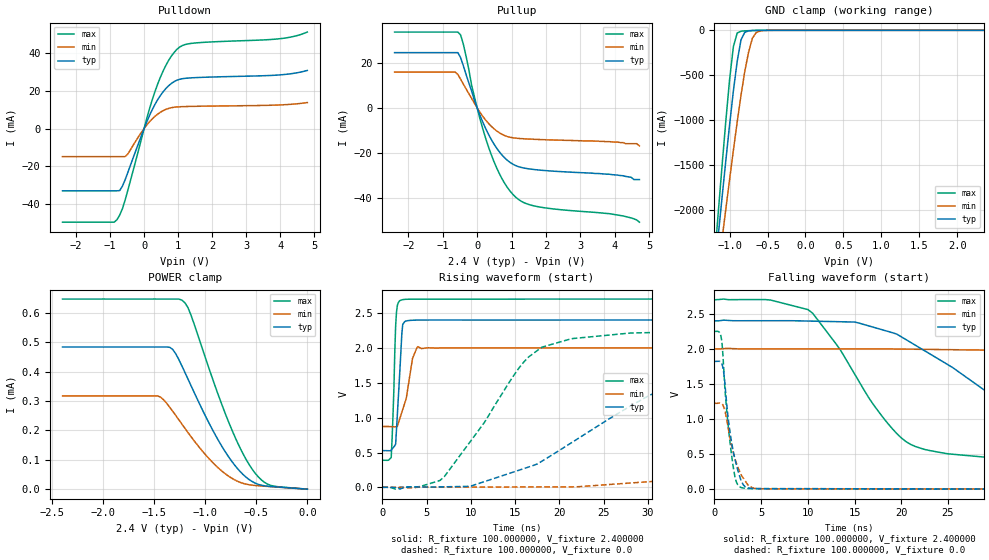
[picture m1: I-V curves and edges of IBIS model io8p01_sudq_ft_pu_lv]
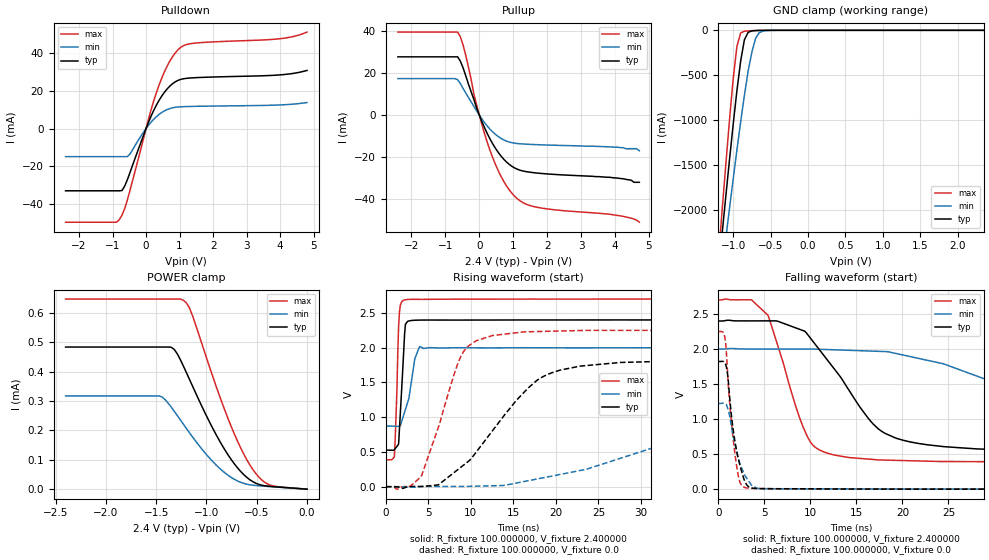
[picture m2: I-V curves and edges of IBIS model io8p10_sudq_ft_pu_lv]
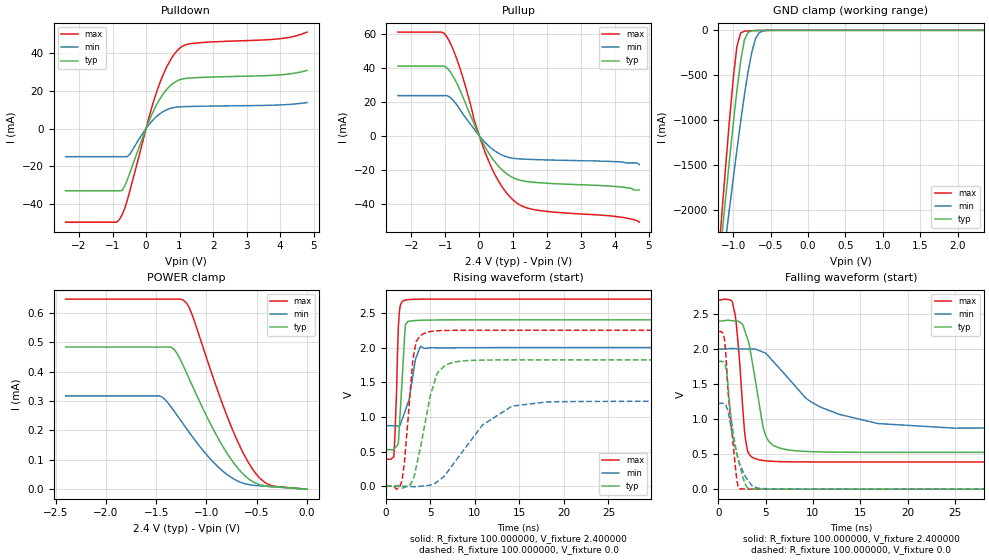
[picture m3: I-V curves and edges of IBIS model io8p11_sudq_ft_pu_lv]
|   stm32f0_444_ufqfpn32 IBIS Model
[IBIS ver]   4.2
[File name]  stm32f0_444_ufqfpn32.ibs
[File Rev]   1.0
[Date]   15-5-2013
[Source] Data Created at STMicroelectronics
[Notes]   File originated from ELDO simulations.
[Disclaimer]  This information is for modeling purpose only and is
   not guaranted. The information is subject to change without
   notice.
[Copyright] Copyright 2015 STMicroelectronics Inc.
[Component] stm32f0_444_ufqfpn32
[Manufacturer] STMicroelectronics
[Package]
| variable   typ   min   max
R_pkg   0.0   NA   NA
L_pkg   0.0H   NA   NA
C_pkg   0.0F   NA   NA
[Pin] signal_name  model_name   R_pin   L_pin   C_pin
0   VSS_VSSA   GND   NA   NA   NA
1   VDD   POWER   0.03449   2.11E-09   6E-14
2   PF0   io8p_sudq_ft   0.029020556   1.54333E-09   3.22222E-14
3   PF1   io8p_sudq_ft   0.025738889   1.20333E-09   1.55556E-14
4   NRST  ioreset_tc_v33   0.024645   1.09E-09   1E-14
5   VDDA  POWER   0.024645   1.09E-09   1E-14
6   PA0   io8p_sudq_ft   0.025738889   1.20333E-09   1.55556E-14
7   PA1   io8p_sudq_ft   0.029020556   1.54333E-09   3.22222E-14
8   PA2   io8p_sudq_ft   0.03449   2.11E-09   6E-14
9   PA3   io8p_sudq_ft   0.03449   2.11E-09   6E-14
10   PA4   io8p_sudq_ft   0.029020556   1.54333E-09   3.22222E-14
11   PA5   io8p_sudq_ft   0.025738889   1.20333E-09   1.55556E-14
12   PA6   io8p_sudq_ft   0.024645   1.09E-09   1E-14
13   PA7   io8p_sudq_ft   0.024645   1.09E-09   1E-14
14   PB0   io8p_sudq_ft   0.025738889   1.20333E-09   1.55556E-14
15   PB1   io8p_sudq_ft   0.029020556   1.54333E-09   3.22222E-14
16   PB2   io8p_sudq_ft   0.03449   2.11E-09   6E-14
17   VDD   POWER   0.03449   2.11E-09   6E-14
18   PA8   io8p_sudq_ft   0.029020556   1.54333E-09   3.22222E-14
19   PA9   io8p_sudq_ft   0.025738889   1.20333E-09   1.55556E-14
20   PA10  io8p_sudq_ft   0.024645   1.09E-09   1E-14
21   PA11  io8p_sudq_ft   0.024645   1.09E-09   1E-14
22   PA12  io8p_sudq_ft   0.025738889   1.20333E-09   1.55556E-14
23   PA13  io8p_sudq_ft   0.029020556   1.54333E-09   3.22222E-14
24   PA14  io8p_sudq_ft   0.03449   2.11E-09   6E-14
25   PA15  io8p_sudq_ft   0.03449   2.11E-09   6E-14
26   PB3   io8p_sudq_ft   0.029020556   1.54333E-09   3.22222E-14
27   PB4   io8p_sudq_ft   0.025738889   1.20333E-09   1.55556E-14
28   PB5   io8p_sudq_ft   0.024645   1.09E-09   1E-14
29   PB6   io8p_sudq_i2cin_lv_ft   0.024645   1.09E-09   1E-14
30   PB7   io8p_sudq_i2cin_lv_ft   0.025738889   1.20333E-09   1.55556E-14
31   BOOT0 vpp_test_hv   0.029020556   1.54333E-09   3.22222E-14
32   PB8   io8p_sudq_i2cin_lv_ft   0.03449   2.11E-09   6E-14
[Model Selector] io8p_sudq_ft
io8p01_sudq_ft_pd_lv  "SPEED01 2P0V, PD=40kOhm"
io8p01_sudq_ft_pu_lv  "SPEED01 2P0V, PU=40kOhm"
io8p01_sudq_ft_lv  "SPEED01 2P0V"
io8p10_sudq_ft_pd_lv  "SPEED10 2P0V, PD=40kOhm"
io8p10_sudq_ft_pu_lv  "SPEED10 2P0V, PU=40kOhm"
io8p10_sudq_ft_lv  "SPEED10 2P0V"
io8p11_sudq_ft_pd_lv  "SPEED11 2P0V, PD=40kOhm"
io8p11_sudq_ft_pu_lv  "SPEED11 2P0V, PU=40kOhm"
io8p11_sudq_ft_lv  "SPEED11 2P0V"
io8p01_sudq_ft_pd  "SPEED01, PD=40kOhm"
io8p01_sudq_ft_pu  "SPEED01, PU=40kOhm"
io8p01_sudq_ft  "SPEED01"
io8p10_sudq_ft_pd  "SPEED10, PD=40kOhm"
io8p10_sudq_ft_pu  "SPEED10, PU=40kOhm"
io8p10_sudq_ft  "SPEED10"
io8p11_sudq_ft_pd  "SPEED11, PD=40kOhm"
io8p11_sudq_ft_pu  "SPEED11, PU=40kOhm"
io8p11_sudq_ft  "SPEED11"
[Model Selector] io8p_sudq_i2cin_lv_ft
io8p01_sudq_i2cin_lv_ft_pd_lv  "SPEED01 2P0V, PD=40kOhm"
io8p01_sudq_i2cin_lv_ft_pu_lv  "SPEED01 2P0V, PU=40kOhm"
io8p01_sudq_i2cin_lv_ft_lv  "SPEED01 2P0V"
io8p10_sudq_i2cin_lv_ft_pd_lv  "SPEED10 2P0V, PD=40kOhm"
io8p10_sudq_i2cin_lv_ft_pu_lv  "SPEED10 2P0V, PU=40kOhm"
io8p10_sudq_i2cin_lv_ft_lv  "SPEED10 2P0V"
io8p11_sudq_i2cin_lv_ft_pd_lv  "SPEED11 2P0V, PD=40kOhm"
io8p11_sudq_i2cin_lv_ft_pu_lv  "SPEED11 2P0V, PU=40kOhm"
io8p11_sudq_i2cin_lv_ft_lv  "SPEED11 2P0V"
io8p01_sudq_i2cin_lv_ft_pd  "SPEED01, PD=40kOhm"
io8p01_sudq_i2cin_lv_ft_pu  "SPEED01, PU=40kOhm"
io8p01_sudq_i2cin_lv_ft  "SPEED01"
io8p10_sudq_i2cin_lv_ft_pd  "SPEED10, PD=40kOhm"
io8p10_sudq_i2cin_lv_ft_pu  "SPEED10, PU=40kOhm"
io8p10_sudq_i2cin_lv_ft  "SPEED10"
io8p11_sudq_i2cin_lv_ft_pd  "SPEED11, PD=40kOhm"
io8p11_sudq_i2cin_lv_ft_pu  "SPEED11, PU=40kOhm"
io8p11_sudq_i2cin_lv_ft  "SPEED11"
[Model Selector] ioreset_tc_v33
ioreset_tc_v33_pu_lv  "IORESET 2V + PU=40kOhm"
ioreset_tc_v33_nopu_lv  "IORESET 2V"
ioreset_tc_v33_pu  "IORESET + PU=40kOhm"
ioreset_tc_v33_nopu  "IORESET"
[Model Selector] vpp_test_hv
vpp_test_hv_3p3  "Input Buffer"
vpp_test_hv_2p4  "Input Buffer 2P0V"
| Models and submodels in the file (42): io8p01_sudq_ft_pd_lv (I/O), io8p01_sudq_ft_pu_lv (I/O), io8p01_sudq_ft_lv (I/O), io8p10_sudq_ft_pd_lv (I/O), io8p10_sudq_ft_pu_lv (I/O), io8p10_sudq_ft_lv (I/O), io8p11_sudq_ft_pd_lv (I/O), io8p11_sudq_ft_pu_lv (I/O), io8p11_sudq_ft_lv (I/O), io8p01_sudq_ft_pd (I/O), io8p01_sudq_ft_pu (I/O), io8p01_sudq_ft (I/O), io8p10_sudq_ft_pd (I/O), io8p10_sudq_ft_pu (I/O), io8p10_sudq_ft (I/O), io8p11_sudq_ft_pd (I/O), io8p11_sudq_ft_pu (I/O), io8p11_sudq_ft (I/O), io8p01_sudq_i2cin_lv_ft_pd_lv (I/O), io8p01_sudq_i2cin_lv_ft_pu_lv (I/O), io8p01_sudq_i2cin_lv_ft_lv (I/O), io8p10_sudq_i2cin_lv_ft_pd_lv (I/O), io8p10_sudq_i2cin_lv_ft_pu_lv (I/O), io8p10_sudq_i2cin_lv_ft_lv (I/O), io8p11_sudq_i2cin_lv_ft_pd_lv (I/O), io8p11_sudq_i2cin_lv_ft_pu_lv (I/O), io8p11_sudq_i2cin_lv_ft_lv (I/O), io8p01_sudq_i2cin_lv_ft_pd (I/O), io8p01_sudq_i2cin_lv_ft_pu (I/O), io8p01_sudq_i2cin_lv_ft (I/O), io8p10_sudq_i2cin_lv_ft_pd (I/O), io8p10_sudq_i2cin_lv_ft_pu (I/O), io8p10_sudq_i2cin_lv_ft (I/O), io8p11_sudq_i2cin_lv_ft_pd (I/O), io8p11_sudq_i2cin_lv_ft_pu (I/O), io8p11_sudq_i2cin_lv_ft (I/O), ioreset_tc_v33_pu_lv (I/O_open_drain), ioreset_tc_v33_nopu_lv (I/O_open_drain), ioreset_tc_v33_pu (I/O_open_drain), ioreset_tc_v33_nopu (I/O_open_drain), vpp_test_hv_2p4 (Input), vpp_test_hv_3p3 (Input)
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|   Model io8p01_sudq_ft_pu_lv
[Model]  io8p01_sudq_ft_pu_lv
Model_type I/O
Polarity   Non-Inverting
Enable   Active-Low
Vinl =   0.720000V
Vinh =   1.680000V
Vmeas =  1.200000V
Cref =   50.000000pF
Rref =   100.000000M
Vref =   0.0V
C_comp   1.970100pF   1.887900pF   2.069400pF
[Temperature Range]   25.000000   0.125000k   -40.000000
[Pullup Reference]   2.400000V   2.000000V   2.700000V
[Pulldown Reference]   0.0V   0.0V   0.0V
[POWER Clamp Reference]   2.400000V   2.000000V   2.700000V
[GND Clamp Reference]   0.0V   0.0V   0.0V
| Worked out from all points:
|   slope of the pulldown table from 0 to 0.36 V, typ, clamps not added: 25.5 ohm
|   slope of the pullup table from 0 to 0.36 V, typ, clamps not added: 28.4 ohm
|   GND clamp passes 1 mA (typ) near -0.64 V on its own axis
|   rising waveform, R_fixture 100.000000, V_fixture 2.400000: 20-80 % time 497ps typ, 1.06ns min, 335ps max; typ from 0.527 V to 2.4 V
|   rising waveform, R_fixture 100.000000, V_fixture 0.0: 20-80 % time 14.6ns typ, 42.8ns min, 7.27ns max; typ from 0.001 V to 1.82 V
|   falling waveform, R_fixture 100.000000, V_fixture 2.400000: 20-80 % time 12.9ns typ, 32.5ns min, 7.06ns max; typ from 2.4 V to 0.527 V
|   falling waveform, R_fixture 100.000000, V_fixture 0.0: 20-80 % time 1.16ns typ, 1.4ns min, 913ps max; typ from 1.82 V to 0.001 V
[Pulldown]
|Voltage   I(typ)   I(min)   I(max)
-2.4V     -33.16mA   -14.98mA   -49.86mA
-880mV    -33.16mA   -14.98mA   -49.86mA
-800mV    -33.16mA   -14.98mA   -48.55mA
-640mV    -30.75mA   -14.98mA   -42.77mA
-480mV    -23.43mA   -13.57mA   -32.92mA
80mV      3.651mA    1.905mA    5.506mA
400mV     15.37mA    7.665mA    23.73mA
720mV     22.75mA    10.69mA    36.23mA
1.04V     26.18mA    11.57mA    43.27mA
1.52V     27.09mA    11.81mA    45.55mA
4V        28.55mA    12.55mA    47.81mA
4.8V      30.9mA     13.81mA    51.31mA
[Pullup]
|Voltage   I(typ)   I(min)   I(max)
-2.4V     24.57mA    15.91mA    33.73mA
-640mV    24.57mA    15.91mA    33.73mA
-480mV    22.32mA    12.71mA    32.43mA
-400mV    18.71mA    10.52mA    28.28mA
-160mV    7.421mA    4.162mA    10.02mA
0V        81fA       15.2pA     0A
320mV     -11.51mA   -6.781mA   -16.98mA
720mV     -21mA      -11.8mA    -31.53mA
1.2V      -26.24mA   -13.65mA   -40.83mA
1.76V     -27.69mA   -14.12mA   -44.07mA
3.84V     -29.6mA    -15.1mA    -47.2mA
4.72V     -32mA      -17mA      -51mA
[GND_clamp]
|Voltage   I(typ)   I(min)   I(max)
-2.4V     -9.788A    -9.782A    -9.734A
-1.2V     -2.718A    -3.02A     -2.568A
-1.15V    -2.29A     -2.675A    -2.036A
-1.1V     -1.868A    -2.333A    -1.515A
-1.05V    -1.454A    -1.995A    -1.012A
-950mV    -674.5mA   -1.337A    -180.5mA
-900mV    -345.2mA   -1.023A    -29.72mA
-850mV    -106.4mA   -726mA     -10.13mA
-750mV    -6.396mA   -244mA     -4.026mA
-700mV    -2.558mA   -88.61mA   -2.329mA
-600mV    -416uA     -7.739mA   -368uA
2.35V     0A         0A         0A
[POWER_clamp]
|Voltage   I(typ)   I(min)   I(max)
-2.4V     483.8uA    317.4uA    647uA
-1.47V    483.8uA    317.4uA    647uA
-1.32V    475.6uA    265.2uA    647uA
-1.23V    419.7uA    221.6uA    643.3uA
-1.17V    374.8uA    192.7uA    617.6uA
-1.14V    352.1uA    178.7uA    591.9uA
-840mV    147uA      62.15uA    289.6uA
-690mV    72.24uA    27.76uA    162.7uA
-540mV    25.74uA    13.55uA    67.63uA
-450mV    13.38uA    10.75uA    31.36uA
-360mV    9.231uA    8.535uA    12.97uA
0V        0A         0A         0A
[Ramp]
| variable   typ   min   max
dV/dt_r  1.09269/14.55881n   0.73353/42.71845n   1.34908/7.26325n
dV/dt_f  1.12400/12.83842n   0.67649/32.44923n   1.38689/7.04961n
R_load = 100.000000
[Rising Waveform]
R_fixture= 100.000000
V_fixture= 2.400000
V_fixture_min= 2.000000
V_fixture_max= 2.700000
|time   V(typ)   V(min)   V(max)
0s        526.5mV    872.5mV    388.6mV
1.001ns   534.8mV    870.7mV    429.3mV
1.301ns   581.8mV    869.1mV    1.401V
1.502ns   620.7mV    868.5mV    2.316V
1.602ns   841mV      868.2mV    2.522V
2.102ns   1.968V     1.038V     2.685V
2.302ns   2.337V     1.118V     2.692V
3.403ns   2.396V     1.846V     2.698V
4.004ns   2.398V     2.018V     2.698V
49.85ns   2.4V       2V         2.7V
[Rising Waveform]
R_fixture= 100.000000
V_fixture= 0.0
V_fixture_min= 0.0
V_fixture_max= 0.0
|time   V(typ)   V(min)   V(max)
0s        1.057mV    1.357mV    941.6uV
6.507ns   6.739mV    4.851mV    98.8mV
15.52ns   249.4mV    5.766mV    1.725V
18.02ns   374.6mV    6.657mV    2.009V
28.03ns   1.166V     62.6mV     2.213V
34.53ns   1.553V     120.9mV    2.23V
43.04ns   1.725V     229mV      2.248V
79.08ns   1.822V     883.8mV    2.25V
103.1ns   1.822V     1.116V     2.249V
249.2ns   1.822V     1.224V     2.25V
[Falling Waveform]
R_fixture= 100.000000
V_fixture= 2.400000
V_fixture_min= 2.000000
V_fixture_max= 2.700000
|time   V(typ)   V(min)   V(max)
0s        2.4V       2V         2.7V
10.01ns   2.397V     2V         2.56V
15.02ns   2.383V     2V         1.64V
20.02ns   2.171V     1.997V     729.2mV
29.53ns   1.353V     1.982V     451.1mV
38.04ns   762.8mV    1.926V     413.2mV
57.06ns   576.4mV    1.555V     391.8mV
84.58ns   537.8mV    1.049V     388.5mV
102.6ns   530.3mV    958.5mV    388.5mV
249.2ns   526.5mV    872.5mV    388.6mV
[Falling Waveform]
R_fixture= 100.000000
V_fixture= 0.0
V_fixture_min= 0.0
V_fixture_max= 0.0
|time   V(typ)   V(min)   V(max)
0s        1.822V     1.224V     2.25V
700.7ps   1.803V     1.224V     2.18V
800.8ps   1.785V     1.217V     2.098V
1.001ns   1.655V     1.167V     1.705V
1.401ns   1.091V     924.7mV    994.1mV
1.802ns   692.7mV    650.1mV    517.8mV
2.302ns   370.4mV    389.6mV    121.1mV
2.903ns   110.3mV    193.7mV    21.86mV
4.605ns   7.762mV    8.133mV    8.175mV
49.85ns   1.057mV    1.357mV    941.6uV
|   Model io8p10_sudq_ft_pu_lv
[Model]  io8p10_sudq_ft_pu_lv
Model_type I/O
Polarity   Non-Inverting
Enable   Active-Low
Vinl =   0.720000V
Vinh =   1.680000V
Vmeas =  1.200000V
Cref =   50.000000pF
Rref =   100.000000M
Vref =   0.0V
C_comp   1.970100pF   1.887900pF   2.069400pF
[Temperature Range]   25.000000   0.125000k   -40.000000
[Pullup Reference]   2.400000V   2.000000V   2.700000V
[Pulldown Reference]   0.0V   0.0V   0.0V
[POWER Clamp Reference]   2.400000V   2.000000V   2.700000V
[GND Clamp Reference]   0.0V   0.0V   0.0V
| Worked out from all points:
|   slope of the pulldown table from 0 to 0.36 V, typ, clamps not added: 25.5 ohm
|   slope of the pullup table from 0 to 0.36 V, typ, clamps not added: 28.4 ohm
|   GND clamp passes 1 mA (typ) near -0.64 V on its own axis
|   rising waveform, R_fixture 100.000000, V_fixture 2.400000: 20-80 % time 500ps typ, 1.06ns min, 335ps max; typ from 0.527 V to 2.4 V
|   rising waveform, R_fixture 100.000000, V_fixture 0.0: 20-80 % time 7.39ns typ, 21.1ns min, 3.53ns max; typ from 0.001 V to 1.82 V
|   falling waveform, R_fixture 100.000000, V_fixture 2.400000: 20-80 % time 6.28ns typ, 17.7ns min, 3.33ns max; typ from 2.4 V to 0.527 V
|   falling waveform, R_fixture 100.000000, V_fixture 0.0: 20-80 % time 1.16ns typ, 1.4ns min, 916ps max; typ from 1.82 V to 0.001 V
[Pulldown]
|Voltage   I(typ)   I(min)   I(max)
-2.4V     -33.16mA   -14.98mA   -49.86mA
-880mV    -33.16mA   -14.98mA   -49.86mA
-800mV    -33.16mA   -14.98mA   -48.55mA
-640mV    -30.75mA   -14.98mA   -42.77mA
-480mV    -23.43mA   -13.57mA   -32.92mA
80mV      3.651mA    1.905mA    5.506mA
400mV     15.37mA    7.665mA    23.73mA
720mV     22.75mA    10.69mA    36.23mA
1.04V     26.18mA    11.57mA    43.27mA
1.52V     27.09mA    11.81mA    45.55mA
4V        28.55mA    12.55mA    47.81mA
4.8V      30.9mA     13.81mA    51.31mA
[Pullup]
|Voltage   I(typ)   I(min)   I(max)
-2.4V     27.74mA    17.38mA    39.53mA
-640mV    27.74mA    16.88mA    39.53mA
-560mV    25.73mA    15.04mA    37.34mA
-480mV    22.58mA    12.74mA    33.42mA
-80mV     3.427mA    2.071mA    4.957mA
160mV     -6.219mA   -3.715mA   -9.137mA
320mV     -11.51mA   -6.781mA   -16.98mA
720mV     -21mA      -11.8mA    -31.53mA
1.12V     -25.77mA   -13.54mA   -39.82mA
1.76V     -27.69mA   -14.12mA   -44.07mA
3.84V     -29.6mA    -15.1mA    -47.2mA
4.72V     -32mA      -17mA      -51mA
[GND_clamp]
|Voltage   I(typ)   I(min)   I(max)
-2.4V     -9.788A    -9.782A    -9.734A
-1.2V     -2.718A    -3.02A     -2.568A
-1.15V    -2.29A     -2.675A    -2.036A
-1.1V     -1.868A    -2.333A    -1.515A
-1.05V    -1.454A    -1.995A    -1.012A
-950mV    -674.5mA   -1.337A    -180.5mA
-900mV    -345.2mA   -1.023A    -29.72mA
-850mV    -106.4mA   -726mA     -10.13mA
-750mV    -6.396mA   -244mA     -4.026mA
-700mV    -2.558mA   -88.61mA   -2.329mA
-600mV    -416uA     -7.739mA   -368uA
2.35V     0A         0A         0A
[POWER_clamp]
|Voltage   I(typ)   I(min)   I(max)
-2.4V     483.8uA    317.4uA    647uA
-1.47V    483.8uA    317.4uA    647uA
-1.32V    475.6uA    265.2uA    647uA
-1.23V    419.7uA    221.6uA    643.3uA
-1.17V    374.8uA    192.7uA    617.6uA
-1.14V    352.1uA    178.7uA    591.9uA
-840mV    147uA      62.15uA    289.6uA
-690mV    72.24uA    27.76uA    162.7uA
-540mV    25.74uA    13.55uA    67.63uA
-450mV    13.38uA    10.75uA    31.36uA
-360mV    9.231uA    8.535uA    12.97uA
0V        0A         0A         0A
[Ramp]
| variable   typ   min   max
dV/dt_r  1.09257/7.38126n   0.73299/21.13981n   1.34920/3.52606n
dV/dt_f  1.12405/6.26972n   0.67519/17.74591n   1.38687/3.32829n
R_load = 100.000000
[Rising Waveform]
R_fixture= 100.000000
V_fixture= 2.400000
V_fixture_min= 2.000000
V_fixture_max= 2.700000
|time   V(typ)   V(min)   V(max)
0s        526.5mV    872.5mV    388.6mV
1.001ns   534.6mV    870.8mV    428.2mV
1.301ns   580.6mV    869.2mV    1.393V
1.502ns   618.8mV    868.6mV    2.312V
1.702ns   1.058V     879.1mV    2.61V
2.102ns   1.96V      1.035V     2.683V
2.302ns   2.337V     1.113V     2.69V
3.403ns   2.395V     1.84V      2.696V
4.004ns   2.398V     2.018V     2.696V
49.85ns   2.4V       2V         2.7V
[Rising Waveform]
R_fixture= 100.000000
V_fixture= 0.0
V_fixture_min= 0.0
V_fixture_max= 0.0
|time   V(typ)   V(min)   V(max)
0s        1.057mV    1.357mV    941.6uV
2.803ns   2.743mV    -4.311mV   6.043mV
4.204ns   4.237mV    2.829mV    160mV
6.206ns   30.25mV    4.308mV    867.3mV
8.809ns   280mV      4.087mV    1.872V
12.61ns   817.4mV    14.56mV    2.176V
17.82ns   1.535V     112.7mV    2.233V
23.02ns   1.737V     237.9mV    2.248V
49.25ns   1.822V     1.075V     2.25V
99.7ns    1.822V     1.224V     2.25V
[Falling Waveform]
R_fixture= 100.000000
V_fixture= 2.400000
V_fixture_min= 2.000000
V_fixture_max= 2.700000
|time   V(typ)   V(min)   V(max)
0s        2.4V       2V         2.7V
3.604ns   2.401V     2V         2.702V
5.405ns   2.402V     2V         2.482V
9.61ns    2.224V     2V         771.1mV
12.61ns   1.714V     1.989V     487.5mV
17.42ns   856.8mV    1.967V     418.1mV
24.42ns   608.6mV    1.79V      395.7mV
43.84ns   535.4mV    1.055V     388.6mV
52.45ns   528.4mV    947.9mV    388.6mV
99.7ns    526.5mV    872.5mV    388.6mV
[Falling Waveform]
R_fixture= 100.000000
V_fixture= 0.0
V_fixture_min= 0.0
V_fixture_max= 0.0
|time   V(typ)   V(min)   V(max)
0s        1.822V     1.224V     2.25V
700.7ps   1.803V     1.224V     2.181V
800.8ps   1.785V     1.216V     2.099V
1.001ns   1.656V     1.167V     1.707V
1.401ns   1.093V     925.2mV    997.9mV
1.902ns   618.4mV    593.3mV    424.7mV
2.302ns   371.4mV    390.6mV    125.2mV
2.903ns   111.3mV    194.4mV    23.9mV
4.705ns   8.256mV    8.438mV    9.524mV
49.85ns   1.057mV    1.357mV    941.6uV
|   Model io8p11_sudq_ft_pu_lv
[Model]  io8p11_sudq_ft_pu_lv
Model_type I/O
Polarity   Non-Inverting
Enable   Active-Low
Vinl =   0.720000V
Vinh =   1.680000V
Vmeas =  1.200000V
Cref =   50.000000pF
Rref =   100.000000M
Vref =   0.0V
C_comp   1.970100pF   1.887900pF   2.069400pF
[Temperature Range]   25.000000   0.125000k   -40.000000
[Pullup Reference]   2.400000V   2.000000V   2.700000V
[Pulldown Reference]   0.0V   0.0V   0.0V
[POWER Clamp Reference]   2.400000V   2.000000V   2.700000V
[GND Clamp Reference]   0.0V   0.0V   0.0V
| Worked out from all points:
|   slope of the pulldown table from 0 to 0.36 V, typ, clamps not added: 25.5 ohm
|   slope of the pullup table from 0 to 0.36 V, typ, clamps not added: 28.4 ohm
|   GND clamp passes 1 mA (typ) near -0.64 V on its own axis
|   rising waveform, R_fixture 100.000000, V_fixture 2.400000: 20-80 % time 508ps typ, 1.05ns min, 337ps max; typ from 0.527 V to 2.4 V
|   rising waveform, R_fixture 100.000000, V_fixture 0.0: 20-80 % time 1.8ns typ, 4.87ns min, 863ps max; typ from 0.001 V to 1.82 V
|   falling waveform, R_fixture 100.000000, V_fixture 2.400000: 20-80 % time 1.39ns typ, 6.08ns min, 775ps max; typ from 2.4 V to 0.527 V
|   falling waveform, R_fixture 100.000000, V_fixture 0.0: 20-80 % time 1.17ns typ, 1.4ns min, 853ps max; typ from 1.82 V to 0.001 V
[Pulldown]
|Voltage   I(typ)   I(min)   I(max)
-2.4V     -33.16mA   -14.98mA   -49.86mA
-880mV    -33.16mA   -14.98mA   -49.86mA
-800mV    -33.16mA   -14.98mA   -48.55mA
-640mV    -30.75mA   -14.98mA   -42.77mA
-480mV    -23.43mA   -13.57mA   -32.92mA
80mV      3.651mA    1.905mA    5.506mA
400mV     15.37mA    7.665mA    23.73mA
720mV     22.75mA    10.69mA    36.23mA
1.04V     26.18mA    11.57mA    43.27mA
1.52V     27.09mA    11.81mA    45.55mA
4V        28.55mA    12.55mA    47.81mA
4.8V      30.9mA     13.81mA    51.31mA
[Pullup]
|Voltage   I(typ)   I(min)   I(max)
-2.4V     41.12mA    23.71mA    61.21mA
-1.12V    41.12mA    23.71mA    61.21mA
-960mV    40.18mA    23.71mA    58.56mA
-800mV    36.01mA    21.55mA    52.29mA
-560mV    26.54mA    15.18mA    39.21mA
-160mV    7.421mA    4.162mA    10.02mA
240mV     -8.977mA   -5.327mA   -13.21mA
640mV     -19.51mA   -11.09mA   -29.16mA
1.04V     -25.15mA   -13.38mA   -38.61mA
1.68V     -27.56mA   -14.07mA   -43.82mA
3.84V     -29.6mA    -15.1mA    -47.2mA
4.72V     -32mA      -17mA      -51mA
[GND_clamp]
|Voltage   I(typ)   I(min)   I(max)
-2.4V     -9.788A    -9.782A    -9.734A
-1.2V     -2.718A    -3.02A     -2.568A
-1.15V    -2.29A     -2.675A    -2.036A
-1.1V     -1.868A    -2.333A    -1.515A
-1.05V    -1.454A    -1.995A    -1.012A
-950mV    -674.5mA   -1.337A    -180.5mA
-900mV    -345.2mA   -1.023A    -29.72mA
-850mV    -106.4mA   -726mA     -10.13mA
-750mV    -6.396mA   -244mA     -4.026mA
-700mV    -2.558mA   -88.61mA   -2.329mA
-600mV    -416uA     -7.739mA   -368uA
2.35V     0A         0A         0A
[POWER_clamp]
|Voltage   I(typ)   I(min)   I(max)
-2.4V     483.8uA    317.4uA    647uA
-1.47V    483.8uA    317.4uA    647uA
-1.32V    475.6uA    265.2uA    647uA
-1.23V    419.7uA    221.6uA    643.3uA
-1.17V    374.8uA    192.7uA    617.6uA
-1.14V    352.1uA    178.7uA    591.9uA
-840mV    147uA      62.15uA    289.6uA
-690mV    72.24uA    27.76uA    162.7uA
-540mV    25.74uA    13.55uA    67.63uA
-450mV    13.38uA    10.75uA    31.36uA
-360mV    9.231uA    8.535uA    12.97uA
0V        0A         0A         0A
[Ramp]
| variable   typ   min   max
dV/dt_r  1.09269/1.79328n   0.73359/4.86832n   1.34926/0.85997n
dV/dt_f  1.12411/1.38607n   0.67669/6.07307n   1.38681/0.77427n
R_load = 100.000000
[Rising Waveform]
R_fixture= 100.000000
V_fixture= 2.400000
V_fixture_min= 2.000000
V_fixture_max= 2.700000
|time   V(typ)   V(min)   V(max)
0s        526.5mV    872.5mV    388.6mV
900.9ps   534.2mV    870.9mV    425.1mV
1.201ns   577.4mV    869.6mV    1.365V
1.401ns   613.7mV    869.2mV    2.295V
1.602ns   1.046V     879.2mV    2.598V
2.202ns   2.333V     1.099V     2.686V
2.603ns   2.381V     1.245V     2.693V
3.303ns   2.389V     1.817V     2.697V
3.904ns   2.394V     2.019V     2.698V
49.85ns   2.4V       2V         2.7V
[Rising Waveform]
R_fixture= 100.000000
V_fixture= 0.0
V_fixture_min= 0.0
V_fixture_max= 0.0
|time   V(typ)   V(min)   V(max)
0s        1.022mV    1.341mV    911uV
1.802ns   -26.21mV   109.9uV    74.5mV
3.103ns   116.7mV    -6.8mV     1.877V
3.403ns   271.6mV    -8.185mV   2.086V
4.505ns   979.1mV    4.99mV     2.215V
5.706ns   1.605V     58.19mV    2.241V
6.707ns   1.752V     167.1mV    2.247V
10.81ns   1.819V     875.7mV    2.25V
14.21ns   1.822V     1.156V     2.25V
49.85ns   1.822V     1.224V     2.25V
[Falling Waveform]
R_fixture= 100.000000
V_fixture= 2.400000
V_fixture_min= 2.000000
V_fixture_max= 2.700000
|time   V(typ)   V(min)   V(max)
0s        2.4V       2V         2.7V
1.502ns   2.403V     2.008V     2.671V
1.902ns   2.401V     2.004V     2.37V
2.903ns   2.224V     2.001V     697.7mV
4.004ns   1.486V     1.995V     432.1mV
5.205ns   712.7mV    1.914V     402.8mV
7.508ns   558.9mV    1.567V     391mV
10.81ns   532.3mV    1.17V      388.6mV
16.82ns   526.7mV    938mV      388.6mV
49.85ns   526.5mV    872.5mV    388.6mV
[Falling Waveform]
R_fixture= 100.000000
V_fixture= 0.0
V_fixture_min= 0.0
V_fixture_max= 0.0
|time   V(typ)   V(min)   V(max)
0s        1.822V     1.224V     2.25V
700.7ps   1.784V     1.216V     2.102V
1.101ns   1.384V     1.072V     1.307V
1.301ns   1.083V     926.1mV    1.012V
1.802ns   627.4mV    595.9mV    327.6mV
2.102ns   434.5mV    435.4mV    35.99mV
2.302ns   325.6mV    349.7mV    5.728mV
3.103ns   17.78mV    137.1mV    2.333mV
4.605ns   2.394mV    9.48mV     1.404mV
49.85ns   1.022mV    1.341mV    911uV
